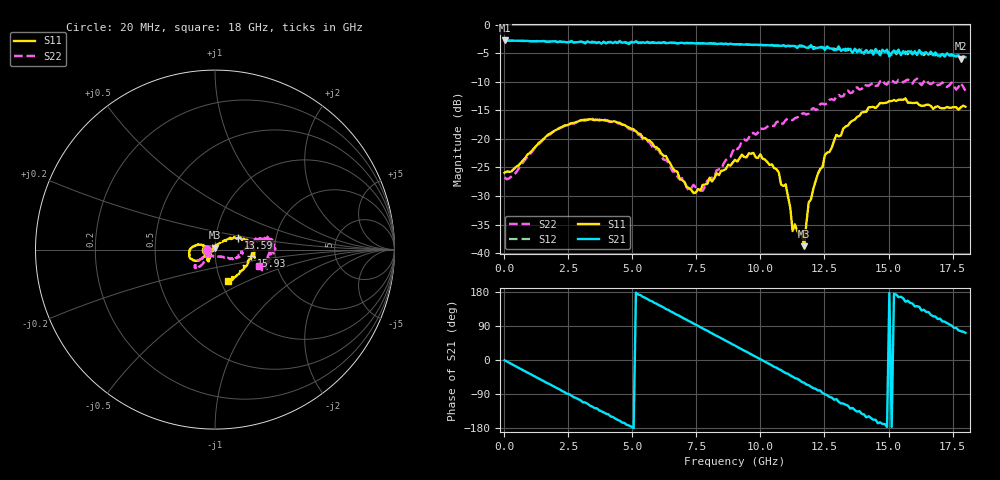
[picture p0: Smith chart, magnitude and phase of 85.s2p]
!Agilent Technologies,N5230A,US43500223,A.07.50.48
!Agilent N5230A: A.07.50.48
!Date: Sunday, January 10, 2016 15:34:55
!Correction: S11(Full 2 Port(1,2))
!S21(Full 2 Port(1,2))
!S12(Full 2 Port(1,2))
!S22(Full 2 Port(1,2))
!S2P File: Measurements: S11, S21, S12, S22:
# Hz S  RI  R 50
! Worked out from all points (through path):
!   201 points, 20 MHz to 18 GHz, reference 50 ohm
!   highest |S21| = -2.76 dB at 20 MHz (marker M1); lowest = -5.9 dB at 17.82 GHz (marker M2)
!   group delay of S21, straight-line fit = 100 ps
!   lowest |S11| = -38.8 dB at 11.71 GHz (marker M3), VSWR 1.02, Z = 50.1 + j1.15 ohm
!   |S11| at or under -10 dB: start of sweep to end of sweep
!   |S22| runs from -29.1 to -9.4 dB; largest |S21 - S12| = 0.075
!   S11 on the Smith chart (normalised r, x): 20 MHz: 0.90, -0.00; 13.59 GHz: 1.28, +0.17; 15.93 GHz: 1.51, -0.11; 18 GHz: 1.08, -0.40
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2e7  -0.0504 -0.000512  0.7277 -0.00949  0.7273 -0.0113  -0.046 -0.00044
1.5483e9  -0.0826 -0.0565  0.4037 -0.5973  0.4006 -0.5963  -0.065 -0.0755
3.0766e9  -0.1387 -0.047  -0.2618 -0.6557  -0.2494 -0.6568  -0.1027 -0.1025
4.515e9  -0.138 0.00464  -0.6717 -0.24  -0.6852 -0.229  -0.1084 -0.0814
6.0433e9  -0.0763 0.027  -0.5689 0.4052  -0.5582 0.4086  -0.0648 -0.0448
7.3918e9  -0.033 -0.0054  -0.0734 0.6849  -0.072 0.6827  -0.00886 -0.0386
7.7514e9  -0.0356 -0.0172  0.0793 0.6832  0.0836 0.6799  0.00545 -0.0347
9.01e9  -0.0334 -0.0564  0.53 0.4157  0.5349 0.4102  0.0681 -0.0487
1.06282e10  -0.0356 -0.041  0.617 -0.2288  0.6114 -0.2373  0.1336 -0.0425
1.09878e10  -0.0251 -0.031  0.5314 -0.3656  0.5359 -0.3675  0.1425 -0.0335
1.12575e10  -0.0125 -0.00924  0.471 -0.4513  0.4668 -0.4532  0.1449 -0.0119
1.1707e10  0.000644 0.0115  0.3222 -0.5584  0.3163 -0.5609  0.1678 -0.000452
1.18868e10  0.00502 0.0273  0.2502 -0.5755  0.245 -0.5922  0.1666 0.00522
1.20666e10  0.0193 0.0311  0.1654 -0.5895  0.1769 -0.6131  0.1859 0.0106
1.29656e10  0.0856 0.0665  -0.1381 -0.5851  -0.1836 -0.577  0.2265 0.0618
1.35949e10  0.1284 0.0662  -0.3355 -0.4549  -0.3827 -0.4529  0.2471 0.0626
1.41343e10  0.1637 0.0554  -0.5267 -0.286  -0.506 -0.3114  0.2913 0.0383
1.50333e10  0.2132 0.0183  -0.526 0.0273  -0.5615 0.0217  0.3202 0.0474
1.59323e10  0.2033 -0.034  -0.4721 0.2814  -0.4639 0.3266  0.3045 0.0059
1.66515e10  0.1671 -0.0988  -0.2807 0.5079  -0.2933 0.4764  0.3013 -0.0082
1.78202e10  0.1029 -0.158  0.121 0.4909  0.1283 0.4957  0.2881 -0.1078
1.8e10  0.0727 -0.1771  0.1614 0.4935  0.1814 0.4871  0.2468 -0.094
